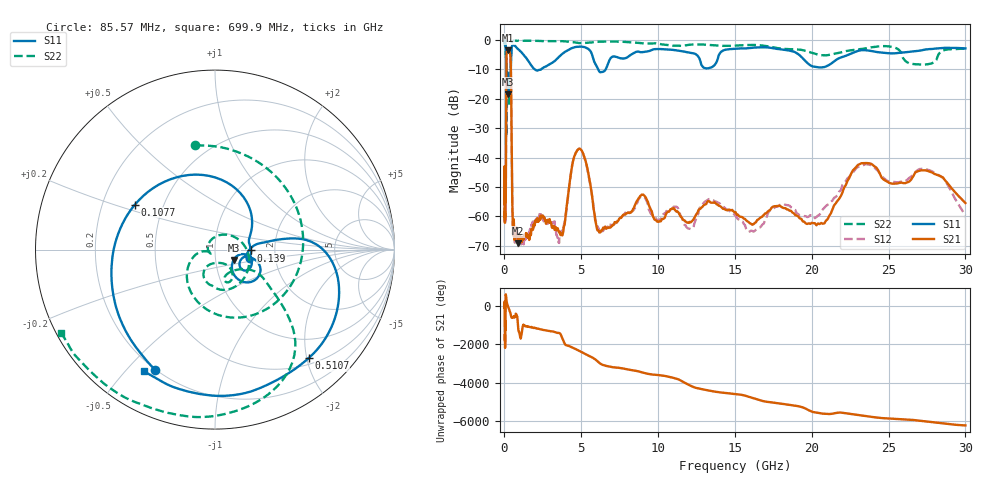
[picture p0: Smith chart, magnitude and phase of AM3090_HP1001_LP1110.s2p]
! Date/Time: Thu, Feb 28, 2019 2:03 PM
! Network Analyzer: Agilent Technologies E8364B Rev: A.07.50.67
! Sweep from 0.010 to 30.000 GHz, 1601 Points, Sweep Type: LOG
! Power Supply: 5.023 V, 0.002 A
# Hz S DB R 50
!freq MagS11 AngS11 MagS21 AngS21 MagS12 AngS12 MagS22 AngS22
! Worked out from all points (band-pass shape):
!   1601 points, 10 MHz to 30 GHz, reference 50 ohm
!   highest |S21| = -3.58 dB at 238.7 MHz (marker M1); lowest = -69.1 dB at 885.5 MHz (marker M2)
!   |S21| within 3 dB of the highest: 126.2 MHz to 399.3 MHz (273.2 MHz wide, 104 % of centre)
!   lowest |S11| = -18.5 dB at 241.1 MHz (marker M3), VSWR 1.27, Z = 61.1 - j7.1 ohm
!   |S11| at or under -10 dB: 119.8 MHz to 414.6 MHz (294.8 MHz wide, 110 % of centre); 1.971 GHz to 2.386 GHz (414.9 MHz wide, 19 % of centre); 6.1 GHz to 6.589 GHz (489.1 MHz wide, 7.71 % of centre)
!   |S22| runs from -32.6 to -0.2 dB; largest |S21 - S12| = 0.011
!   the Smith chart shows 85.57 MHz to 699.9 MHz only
!   S11 on the Smith chart (normalised r, x): 85.57 MHz: 0.20, -0.60; 107.7 MHz: 0.34, +0.23; 139 MHz: 1.50, -0.02; 510.7 MHz: 0.61, -2.04; 699.9 MHz: 0.16, -0.56
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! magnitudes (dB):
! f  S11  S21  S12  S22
! 10 MHz  -0.3  -43.1  -42.8  -0.7
! 38.04 MHz  -0.5  -59.9  -60.2  -1.6
! 85.57 MHz  -2.5  -53.7  -56.7  -4.6
! 107.7 MHz  -5.8  -23.9  -23.9  -6.6
! 139 MHz  -13.9  -4.8  -4.7  -30.1
! 144.7 MHz  -14.0  -4.4  -4.4  -28.2
! 238.7 MHz  -18.4  -3.6  -3.6  -13.9
! 241.1 MHz  -18.5  -3.6  -3.6  -13.9
! 309.6 MHz  -15.5  -3.8  -3.7  -22.5
! 405.7 MHz  -11.2  -7.3  -7.3  -8.9
! 510.7 MHz  -2.0  -55.1  -56.1  -0.5
! 550.5 MHz  -1.9  -64.2  -62.8  -0.4
! 699.9 MHz  -2.1  -66.1  -66.9  -0.2
! 885.5 MHz  -3.1  -69.1  -69.0  -0.3
! 2.084 GHz  -10.4  -61.4  -60.9  -0.3
! 3.613 GHz  -5.5  -65.6  -66.7  -0.5
! 4.854 GHz  -2.3  -37.0  -37.0  -1.1
! 6.141 GHz  -10.4  -64.9  -64.2  -0.6
! 7.926 GHz  -6.1  -59.0  -58.4  -0.7
! 20.2 GHz  -9.2  -62.3  -60.6  -4.7
! 23.48 GHz  -3.5  -41.9  -42.2  -2.9
! 30 GHz  -2.9  -55.4  -59.6  -3.0
